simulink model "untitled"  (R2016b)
settings: Solver=FixedStepDiscrete  StartTime=0.0  StopTime=10.0  RelTol=1e-3  EnableMultiTasking=on
libraries: c2837xDlib x2, c280xlib x1

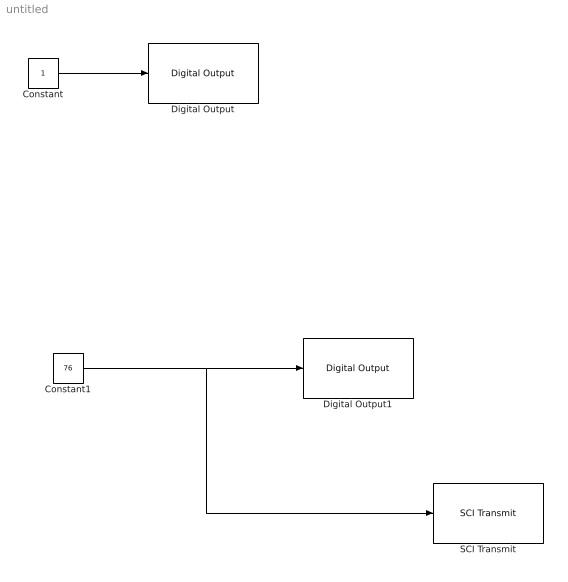
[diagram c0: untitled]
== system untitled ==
  Constant : Constant  OutDataTypeStr=uint16  SampleTime=0.05
  Constant1 : Constant  Value=76  OutDataTypeStr=uint16  SampleTime=1.5
  Digital Output : c2837xDlib/Digital Output  GPIO_Number=GPIO32~GPIO39  GPIO_Bit0=off  GPIO_BIT0_Toggle=off  GPIO_Bit1=off  GPIO_BIT1_Toggle=off  GPIO_Bit2=on  GPIO_BIT2_Toggle=on  GPIO_Bit3=off  GPIO_BIT3_Toggle=off  GPIO_Bit4=off  GPIO_BIT4_Toggle=off  GPIO_Bit5=off  GPIO_BIT5_Toggle=off  GPIO_Bit6=off  GPIO_BIT6_Toggle=off  GPIO_Bit7=off  GPIO_BIT7_Toggle=off
  Digital Output1 : c2837xDlib/Digital Output  GPIO_Number=GPIO24~GPIO31  GPIO_Bit0=off  GPIO_BIT0_Toggle=off  GPIO_Bit1=off  GPIO_BIT1_Toggle=off  GPIO_Bit2=off  GPIO_BIT2_Toggle=on  GPIO_Bit3=off  GPIO_BIT3_Toggle=off  GPIO_Bit4=off  GPIO_BIT4_Toggle=off  GPIO_Bit5=off  GPIO_BIT5_Toggle=off  GPIO_Bit6=off  GPIO_BIT6_Toggle=off  GPIO_Bit7=on  GPIO_BIT7_Toggle=on
  SCI Transmit : c280xlib/SCI Transmit  sciModule=A  dataHead=''  dataTail=''  postInterrupt=off  numFifo=1
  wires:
  Constant/1 -> Digital Output/1
  Constant1/1 -> SCI Transmit/1, Digital Output1/1
